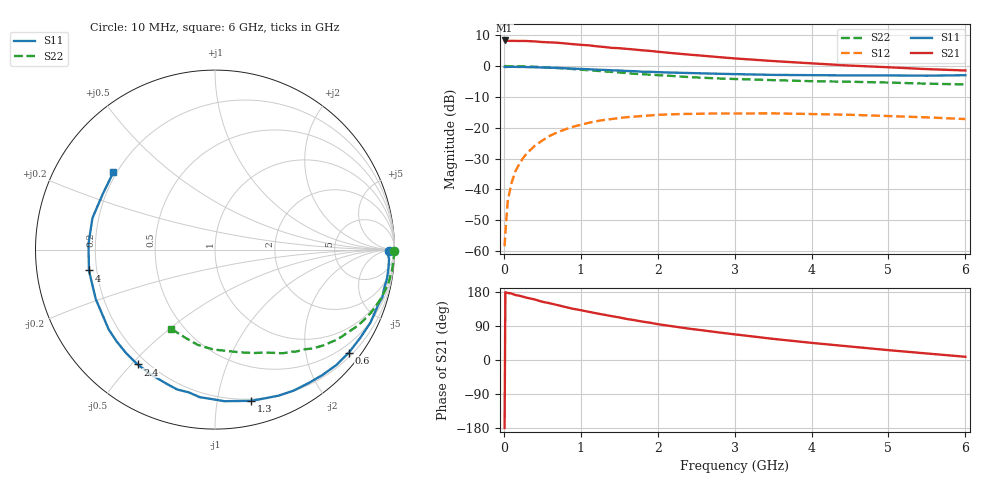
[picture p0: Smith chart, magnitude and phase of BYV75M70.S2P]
! SIEMENS Small Signal Semiconductors
! BFY420
! Si NPN RF SIEGET Grounded Emitter Transistor in MICRO-X
! VCE = 0.75 V  IC = 0.7 mA
! Common Emitter S-Parameters:  October  1996
# GHz  S  MA  R  50
!  f  S11  S21  S12  S22
! GHz  MAG  ANG  MAG  ANG  MAG  ANG  MAG  ANG
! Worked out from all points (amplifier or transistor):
!   36 points, 10 MHz to 6 GHz, reference 50 ohm
!   highest |S21| = 8.3 dB at 10 MHz (marker M1)
!   |S21| within 3 dB of that: start of sweep to 1.721 GHz
!   unconditionally stable (mu >= 1): 4.686 GHz to end of sweep
!   at 250 MHz: K = 0.04, MSG = 19.0 dB, |S12| = -29.9 dB
!   at 1.4 GHz: K = 0.23, MSG = 11.6 dB, |S12| = -17.2 dB
!   at 6 GHz: K = 1.34, MAG = 4.4 dB, |S12| = -17.2 dB
!   S11 on the Smith chart (normalised r, x): 10 MHz: 62, -23; 600 MHz: 0.29, -2.91; 1.3 GHz: 0.19, -1.25; 2.4 GHz: 0.16, -0.52; 4 GHz: 0.17, -0.08; 6 GHz: 0.19, +0.33
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0.01  0.9721 -0.6  2.602 -179.3  0.0012 104.6  0.9987 -0.3
0.02  0.9632 -1.6  2.598 178.8  0.002 82.9  0.9999 -0.7
0.05  0.9713 -3.1  2.568 177.0  0.0064 88.6  0.9976 -1.7
0.1  0.9723 -6.4  2.559 175.3  0.0127 86.2  0.9953 -3.5
0.15  0.9718 -9.6  2.56 171.5  0.0196 82.9  0.9937 -5.3
0.3  0.9598 -18.8  2.546 164.2  0.0386 77.8  0.9856 -10.4
0.4  0.9569 -25.2  2.511 159.8  0.0507 73.4  0.9737 -13.8
0.5  0.9468 -31.3  2.452 153.7  0.0621 69.4  0.9607 -17.1
0.6  0.9412 -37.6  2.422 149.6  0.0742 65.6  0.9461 -20.3
0.8  0.9201 -49.4  2.327 139.8  0.0945 57.6  0.9115 -26.4
1.1  0.8877 -66.4  2.173 127.3  0.12 47.1  0.8565 -34.5
1.3  0.8665 -76.5  2.043 119.6  0.1336 40.9  0.8213 -39.3
1.7  0.8267 -95.9  1.853 105.1  0.1516 29.7  0.7492 -47.8
2  0.7962 -109.2  1.708 94.6  0.1616 22.6  0.7117 -53.1
2.2  0.7827 -116.8  1.617 88.7  0.1655 18.0  0.6901 -56.8
2.4  0.7717 -124.0  1.537 82.9  0.1676 14.4  0.6638 -60.1
2.8  0.7496 -137.1  1.395 72.6  0.1707 7.5  0.6286 -66.1
3.5  0.7193 -157.5  1.206 55.8  0.171 -2.1  0.5912 -75.7
4  0.7119 -170.6  1.107 45.2  0.1668 -8.0  0.5689 -83.2
4.5  0.7055 177.4  1.019 35.6  0.162 -13.3  0.5567 -90.8
5.5  0.6979 153.5  0.892 17.2  0.1472 -20.2  0.5181 -108.8
6  0.7113 142.8  0.848 8.5  0.1383 -21.6  0.5038 -118.9
